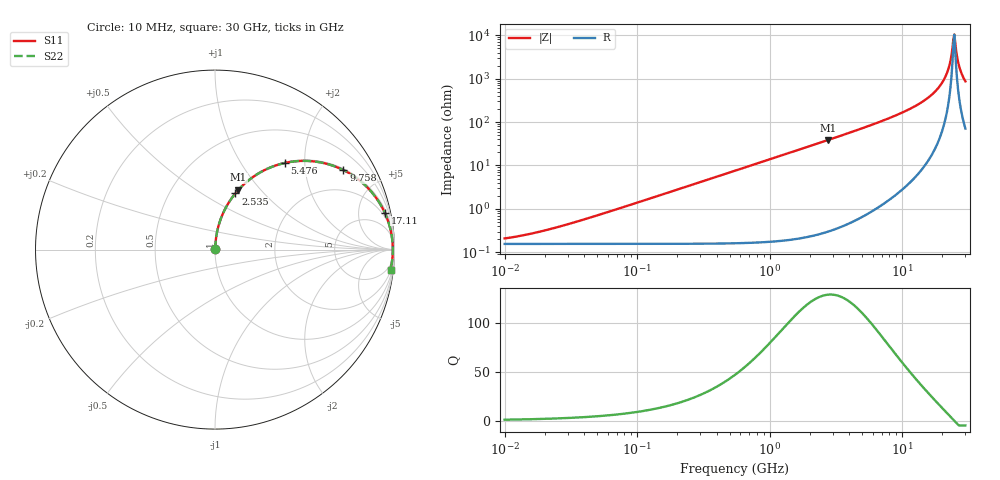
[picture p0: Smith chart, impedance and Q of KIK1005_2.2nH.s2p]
!version-3
!date-01.2023
!Series
# Hz S RI R 50
!Freq ReS11 ImS11 ReS21 ImS21 ReS12 ImS12 ReS22 ImS22
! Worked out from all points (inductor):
!   500 points, 10 MHz to 30 GHz, reference 50 ohm
!   read as one part in series: L = 2.2 nH near 33.85 MHz
!   highest Q = 129 at 2.747 GHz (marker M1), where L = 2.23 nH
!   self-resonance near 24.35 GHz
!   S11 on the Smith chart (normalised r, x): 10 MHz: 1.00, +0.00; 2.535 GHz: 1.01, +0.71; 5.476 GHz: 1.02, +1.59; 9.758 GHz: 1.05, +3.20; 17.11 GHz: 1.40, +9.09; 30 GHz: 2, -17
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1e7  0.00156 0.00138  0.9984 -0.00138  0.9984 -0.00138  0.00156 0.00138
3.848815e7  0.00158 0.0053  0.9984 -0.0053  0.9984 -0.0053  0.00158 0.0053
1.457759e8  0.00196 0.0201  0.998 -0.0201  0.998 -0.0201  0.00196 0.0201
5.521343e8  0.00738 0.0757  0.9926 -0.0757  0.9926 -0.0757  0.00738 0.0757
2.091238e9  0.08 0.2672  0.92 -0.2672  0.92 -0.2672  0.08 0.2672
2.535255e9  0.1134 0.3132  0.8866 -0.3132  0.8866 -0.3132  0.1134 0.3132
2.747025e9  0.1307 0.3332  0.8693 -0.3332  0.8693 -0.3332  0.1307 0.3332
5.476389e9  0.389 0.4827  0.611 -0.4827  0.611 -0.4827  0.389 0.4827
7.920679e9  0.5971 0.484  0.4029 -0.484  0.4029 -0.484  0.5971 0.484
9.757729e9  0.7156 0.4431  0.2844 -0.4431  0.2844 -0.4431  0.7156 0.4431
1.344969e10  0.8685 0.3253  0.1315 -0.3253  0.1315 -0.3253  0.8685 0.3253
1.710941e10  0.9457 0.2057  0.0543 -0.2057  0.0543 -0.2057  0.9457 0.2057
1.945272e10  0.9716 0.1356  0.0284 -0.1356  0.0284 -0.1356  0.9716 0.1356
2.141852e10  0.9839 0.0813  0.0161 -0.0813  0.0161 -0.0813  0.9839 0.0813
2.247471e10  0.9877 0.0538  0.0123 -0.0538  0.0123 -0.0538  0.9877 0.0538
2.320761e10  0.9893 0.0354  0.0107 -0.0354  0.0107 -0.0354  0.9893 0.0354
2.396441e10  0.9903 0.017  0.00968 -0.017  0.00968 -0.017  0.9903 0.017
2.474589e10  0.9906 -0.00149  0.00938 0.00149  0.00938 0.00149  0.9906 -0.00149
2.514614e10  0.9905 -0.0107  0.00949 0.0107  0.00949 0.0107  0.9905 -0.0107
2.638614e10  0.9891 -0.0384  0.0109 0.0384  0.0109 0.0384  0.9891 -0.0384
2.724659e10  0.9874 -0.0568  0.0126 0.0568  0.0126 0.0568  0.9874 -0.0568
3e10  0.9779 -0.1115  0.0221 0.1115  0.0221 0.1115  0.9779 -0.1115
